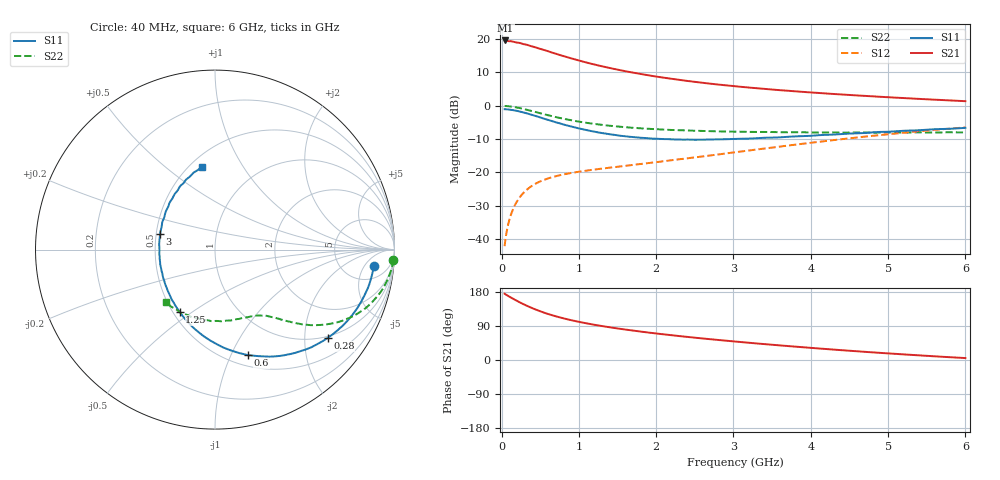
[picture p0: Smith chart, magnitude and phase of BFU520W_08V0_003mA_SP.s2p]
! Filename:  P:\Prog\Test\Noise\ATS_data\Testdata_Net\Run2\BFU520W_APM2013_06_A05_08p0V_003mA_SP_CM01_D.s2p
! Date/Time: Tue 26/Mar/2013 18:01:42
! BFU520W_APM2013_06_A05_08p0V_1to20mA_SP_CM01_Bias3_R.s2p
! MDIF S-parameter v. bias file
! BFU520W_APM2013_06_A05_08p0V_1to20mA_SP_CM01
! Date/time Thu Mar 21 15:28:29 2013
! VAR V_out= 8.0000
! VAR I_out= 3.0000
! VAR V_in= 0.8141
! VAR I_in= 0.0324
! Device data file deembeded for feedlines and parallel
! Original file: \Run2\BFU520W_APM2013_06_A05_08p0V_003mA_SP_CM01_R.s2p
! Feed-files: PR019V01_070313_Feed1.s2p, PR019V01_070313_Feed2.s2p
! Parallel-file: PR019V01_070313_Par.s2p
# MHz S MA R 50
!  Freq-MHz  S11-mag  S11-arg  S21-mag  S21-arg  S12-mag  S12-arg  S22-mag  S22-arg
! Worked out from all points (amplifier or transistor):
!   98 points, 40 MHz to 6 GHz, reference 50 ohm
!   highest |S21| = 19.6 dB at 50 MHz (marker M1)
!   |S21| within 3 dB of that: start of sweep to 570 MHz
!   unconditionally stable (mu >= 1): 2.162 GHz to 3.282 GHz
!   at 300 MHz: K = 0.23, MSG = 22.1 dB, |S12| = -25.8 dB
!   at 1.6 GHz: K = 0.89, MSG = 14.2 dB, |S12| = -18.0 dB
!   at 6 GHz: K = 0.84, MSG = 3.9 dB, |S12| = -6.5 dB
!   S11 on the Smith chart (normalised r, x): 40 MHz: 10, -8; 280 MHz: 0.96, -2.59; 600 MHz: 0.61, -1.16; 1.25 GHz: 0.54, -0.45; 3 GHz: 0.52, +0.10; 6 GHz: 0.57, +0.68
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40  0.8894 -5.7  9.543 174.9  0.007829 85.9  0.9949 -3.3
50  0.8889 -7.1  9.569 173.4  0.009737 85.4  0.9929 -4.1
60  0.8868 -8.6  9.443 172.2  0.01166 84.8  0.9921 -5.0
120  0.8708 -17.1  9.328 165.0  0.02289 80.0  0.9765 -9.8
160  0.8566 -22.6  9.118 160.5  0.03007 76.9  0.9617 -12.9
240  0.8183 -33.2  8.746 151.7  0.04296 71.4  0.9224 -18.6
280  0.7978 -38.1  8.458 147.7  0.04881 68.9  0.9008 -21.2
340  0.7637 -45.5  8.158 142.0  0.05661 65.6  0.8651 -24.7
420  0.7157 -54.5  7.656 134.9  0.06574 61.8  0.819 -28.6
500  0.6695 -63.0  7.16 128.7  0.07338 58.7  0.7745 -32.0
600  0.6159 -72.6  6.61 121.6  0.08121 55.7  0.7229 -35.5
700  0.5673 -81.3  6.065 115.4  0.08772 53.5  0.6788 -38.3
800  0.5254 -89.2  5.581 110.0  0.09324 51.9  0.6407 -40.5
1050  0.4454 -107.0  4.62 98.7  0.1044 50.1  0.5667 -44.7
1250  0.399 -119.5  4.042 91.2  0.1124 49.8  0.5263 -47.2
1600  0.3494 -138.9  3.311 80.4  0.1257 51.0  0.4783 -51.1
2050  0.3187 -160.1  2.694 68.8  0.1451 53.5  0.4425 -56.0
3000  0.318 164.2  1.979 49.1  0.1996 57.2  0.4094 -69.3
3100  0.3205 160.9  1.927 47.3  0.2064 57.3  0.4087 -70.8
4100  0.3624 134.7  1.561 30.5  0.2879 55.7  0.3974 -89.2
5200  0.4219 112.5  1.308 14.8  0.3946 48.5  0.3954 -113.1
6000  0.4666 99.0  1.174 5.1  0.4741 41.1  0.3985 -132.8
